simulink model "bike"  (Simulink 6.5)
settings: Solver=ode45  StartTime=0.0  StopTime=10.0  MaxStep=0.01  RelTol=1e-3
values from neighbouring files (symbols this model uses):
  K = [K zeros(2, 2)]    [designLQR.m]    (also in mc_approx.m = reshape(K, N0); mc_approx_vectorized.m = reshape(K, N0); end; genmpc_exp.m = find(~isnan(e_R(1, :, trial)), 1, 'last') - 1; qlearn_exp.m = find(~isnan(e_R(1, :, trial)), 1, 'last'))
libraries: simulink x3

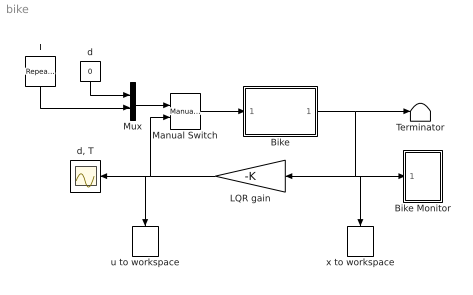
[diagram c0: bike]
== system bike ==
  Bike : Subsystem
  Bike Monitor : Subsystem
  LQR gain : Gain  Orientation=left  Gain=-K  Multiplication=Matrix(K*u) (u vector)
  Manual Switch : simulink/Signal Routing/Manual Switch  SystemSampleTime=-1  sw=0  action=0
  Mux : Mux  Inputs=2
  T : simulink/Sources/Repeating Sequence  Orientation=down  SystemSampleTime=-1  rep_seq_t=[0 1 1 1e10]  rep_seq_y=[0 .001 0 0]
  Terminator : Terminator
  d : Constant  Orientation=down  Value=0  OutDataType=sfix(16)  ConRadixGroup=Use specified scaling  OutScaling=2^0  SampleTime=inf  FramePeriod=inf
  "d, T" : Scope
  u to workspace : ToWorkspace  VariableName=simu  SampleTime=-1  SaveFormat=Structure With Time
  x to workspace : ToWorkspace  VariableName=simx  SampleTime=-1  SaveFormat=Structure With Time
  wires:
  Bike/1(x) -> Terminator/1, Bike Monitor/1(x), LQR gain/1, x to workspace/1
  d/1 -> Mux/1
  T/1 -> Mux/2
  Mux/1 -> Manual Switch/1
  Manual Switch/1 -> Bike/1(u)
  LQR gain/1 -> Manual Switch/2, "d, T"/1, u to workspace/1

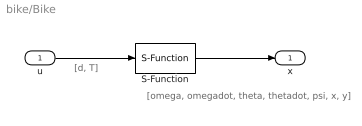
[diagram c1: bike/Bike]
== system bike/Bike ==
  note: [d, T]
  note: [omega, omegadot, theta, thetadot, psi, x, y]
  u : Inport
  S-Function : S-Function  FunctionName=bike_sfun
  x : Outport
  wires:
  u/1 -> S-Function/1
  S-Function/1 -> x/1

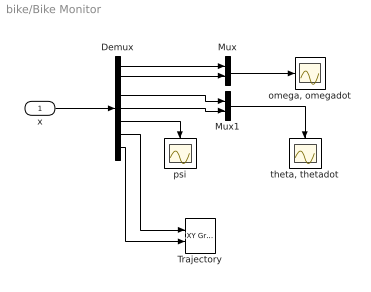
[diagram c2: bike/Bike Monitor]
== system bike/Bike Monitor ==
  x : Inport
  Demux : Demux  Outputs=7
  Mux : Mux  Inputs=2
  Mux1 : Mux  Inputs=2
  Trajectory : simulink/Sinks/XY Graph  SystemSampleTime=-1  xmin=-50  xmax=50  ymin=-50  ymax=50  st=-1
  "omega, omegadot" : Scope
  psi : Scope
  "theta, thetadot" : Scope
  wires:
  x/1 -> Demux/1
  Demux/1 -> Mux/1
  Demux/2 -> Mux/2
  Mux/1 -> "omega, omegadot"/1
  Demux/3 -> Mux1/1
  Demux/4 -> Mux1/2
  Mux1/1 -> "theta, thetadot"/1
  Demux/7 -> Trajectory/2
  Demux/6 -> Trajectory/1
  Demux/5 -> psi/1
